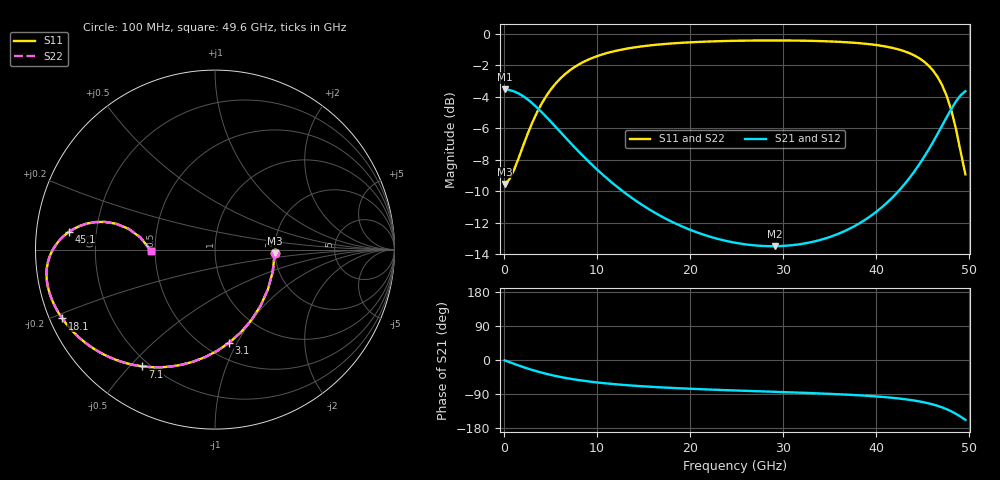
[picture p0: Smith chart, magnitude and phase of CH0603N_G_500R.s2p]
# GHz S RI R 500
! S-Parameters data
! Freq  reS11  imS11  reS21  imS21  reS12  imS12  reS22  imS22
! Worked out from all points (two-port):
!   100 points, 100 MHz to 49.6 GHz, reference 500 ohm
!   highest |S21| = -3.52 dB at 100 MHz (marker M1); lowest = -13.5 dB at 29.1 GHz (marker M2)
!   |S21| within 3 dB of the highest: start of sweep to 6.541 GHz; 46.45 GHz to end of sweep
!   lowest |S11| = -9.5 dB at 100 MHz (marker M3), VSWR 2.00, Z = 998 - j46.6 ohm
!   |S11| at or under -10 dB: nowhere
!   |S22| runs from -9.5 to -0.4 dB; largest |S21 - S12| = 0
!   S11 on the Smith chart (normalised r, x): 100 MHz: 2.00, -0.09; 3.1 GHz: 0.65, -0.93; 7.1 GHz: 0.17, -0.54; 18.1 GHz: 0.04, -0.21; 45.1 GHz: 0.10, +0.06; 49.6 GHz: 0.47, -0.01
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0.1  0.333 -0.0207  0.6665 -0.0107  0.6665 -0.0107  0.333 -0.0207
0.6  0.3216 -0.1233  0.6607 -0.0635  0.6607 -0.0635  0.3216 -0.1233
1.6  0.2544 -0.312  0.6267 -0.1608  0.6267 -0.1608  0.2544 -0.312
3.1  0.0787 -0.519  0.538 -0.2683  0.538 -0.2683  0.0787 -0.519
4.1  -0.0564 -0.5996  0.47 -0.3109  0.47 -0.3109  -0.0564 -0.5996
5.1  -0.1864 -0.6417  0.4046 -0.3342  0.4046 -0.3342  -0.1864 -0.6417
7.1  -0.4042 -0.6508  0.2955 -0.3433  0.2955 -0.3433  -0.4042 -0.6508
8.6  -0.5264 -0.6232  0.2344 -0.3332  0.2344 -0.3332  -0.5264 -0.6232
10.1  -0.6193 -0.5845  0.1879 -0.3177  0.1879 -0.3177  -0.6193 -0.5845
12.1  -0.7093 -0.5287  0.1429 -0.2954  0.1429 -0.2954  -0.7093 -0.5287
16.6  -0.8269 -0.4156  0.0834 -0.2531  0.0834 -0.2531  -0.8269 -0.4156
18.1  -0.8508 -0.3835  0.071 -0.2425  0.071 -0.2425  -0.8508 -0.3835
25.1  -0.9144 -0.2632  0.0353 -0.2134  0.0353 -0.2134  -0.9144 -0.2632
29.1  -0.931 -0.2072  0.0223 -0.2103  0.0223 -0.2103  -0.931 -0.2072
33.1  -0.9384 -0.1531  0.00971 -0.2178  0.00971 -0.2178  -0.9384 -0.1531
37.6  -0.934 -0.0852  -0.0102 -0.2439  -0.0102 -0.2439  -0.934 -0.0852
41.6  -0.9054 -0.00425  -0.0488 -0.2948  -0.0488 -0.2948  -0.9054 -0.00425
45.1  -0.8134 0.0989  -0.1475 -0.3757  -0.1475 -0.3757  -0.8134 0.0989
46.6  -0.7169 0.1441  -0.2465 -0.4124  -0.2465 -0.4124  -0.7169 0.1441
48.1  -0.552 0.1443  -0.4136 -0.4044  -0.4136 -0.4044  -0.552 0.1443
49.1  -0.4152 0.0675  -0.5517 -0.3225  -0.5517 -0.3225  -0.4152 0.0675
49.6  -0.3578 -0.00588  -0.6098 -0.2467  -0.6098 -0.2467  -0.3578 -0.00588
